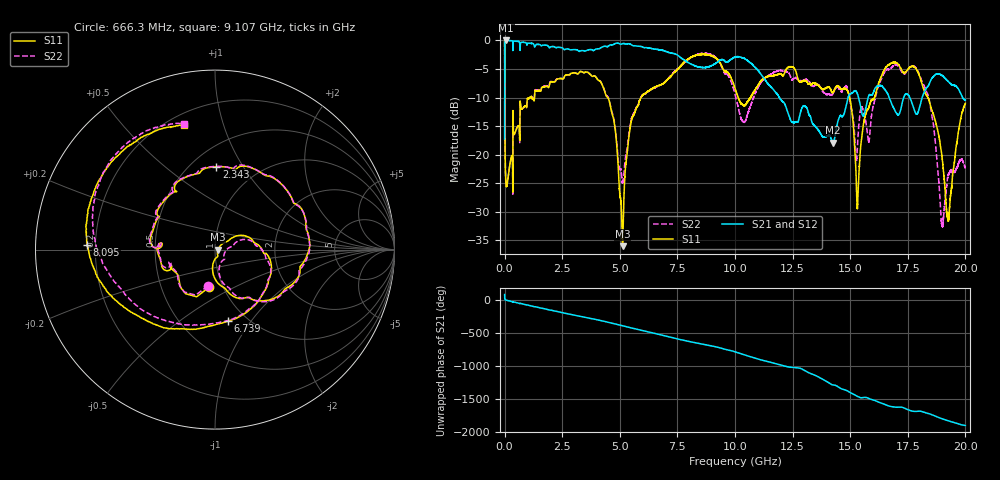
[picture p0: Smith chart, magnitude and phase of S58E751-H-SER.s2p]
!{S58E751}
!Johanson Technology Inc.
!www.johansontechnology.com
!Test Board Conditions:
!Substrate Type  RO4350B
!Substrate Thickness  60 mil
!Substrate Dk  3.66
!TL Type: GCPW
!TL Trace Width  115 mil
!TL Gap  52 mil
!Electrode orientation  Horizontal
!DUT TOPOLOGY	SERIES
!Mounting Pad LxW  55x428 mil
! Created Wed Apr 14 12:02:31 2021
# mhz S ma R 50
! 2 Port Network Data from SP1.SP block
! freq  magS11  angS11  magS21  angS21  magS12  angS12  magS22  angS22
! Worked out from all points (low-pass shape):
!   20001 points, 300 kHz to 20 GHz, reference 50 ohm
!   highest |S21| = -0.01 dB at 72.3 MHz (marker M1); lowest = -17.9 dB at 14.26 GHz (marker M2)
!   |S21| within 3 dB of the highest: 2.216 MHz to 7.64 GHz (7.637 GHz wide, 200 % of centre); 9.948 GHz to 10.29 GHz (339.9 MHz wide, 3.36 % of centre)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
!   lowest |S11| = -36.0 dB at 5.126 GHz (marker M3), VSWR 1.03, Z = 51.6 - j0.0582 ohm
!   |S11| at or under -10 dB: 6.522 MHz to 1.099 GHz (1.093 GHz wide, 198 % of centre); 4.479 GHz to 5.922 GHz (1.443 GHz wide, 27.8 % of centre); 18.37 GHz to end of sweep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
!   |S22| runs from -32.7 to -0.1 dB; largest |S21 - S12| = 0.013
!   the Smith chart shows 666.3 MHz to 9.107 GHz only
!   S11 on the Smith chart (normalised r, x): 666.3 MHz: 0.86, -0.38; 2.343 GHz: 0.66, +0.77; 6.739 GHz: 0.82, -0.78; 8.095 GHz: 0.17, +0.02; 9.107 GHz: 0.26, +0.75
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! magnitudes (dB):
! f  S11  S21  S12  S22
! 300 kHz  -0.1  -17.2  -17.2  -0.1
! 72.3 MHz  -25.5  0.0  0.0  -25.4
! 666.3 MHz  -13.4  -1.6  -1.6  -13.7
! 2.343 GHz  -6.7  -1.2  -1.2  -6.7
! 3.334 GHz  -5.5  -1.8  -1.8  -5.5
! 4.549 GHz  -10.7  -0.9  -0.9  -10.6
! 5.126 GHz  -36.0  -0.6  -0.5  -25.0
! 5.54 GHz  -13.5  -0.9  -0.8  -13.2
! 6.667 GHz  -7.9  -1.6  -1.6  -7.9
! 6.739 GHz  -7.8  -1.7  -1.7  -7.8
! 8.095 GHz  -2.9  -4.2  -4.1  -3.0
! 9.107 GHz  -2.9  -4.1  -4.2  -2.8
! 10 GHz  -8.4  -2.9  -2.9  -9.5
! 13.33 GHz  -7.6  -14.3  -14.2  -8.0
! 14.26 GHz  -9.1  -17.9  -17.8  -9.3
! 14.95 GHz  -9.6  -9.6  -9.7  -9.7
! 15.32 GHz  -28.7  -9.5  -9.5  -17.9
! 16.67 GHz  -4.3  -9.7  -9.8  -5.1
! 17.98 GHz  -6.0  -12.1  -12.1  -5.8
! 18.98 GHz  -20.1  -6.1  -6.1  -32.0
! 19.24 GHz  -31.3  -7.1  -7.1  -23.9
! 20 GHz  -11.0  -10.4  -10.3  -22.5
